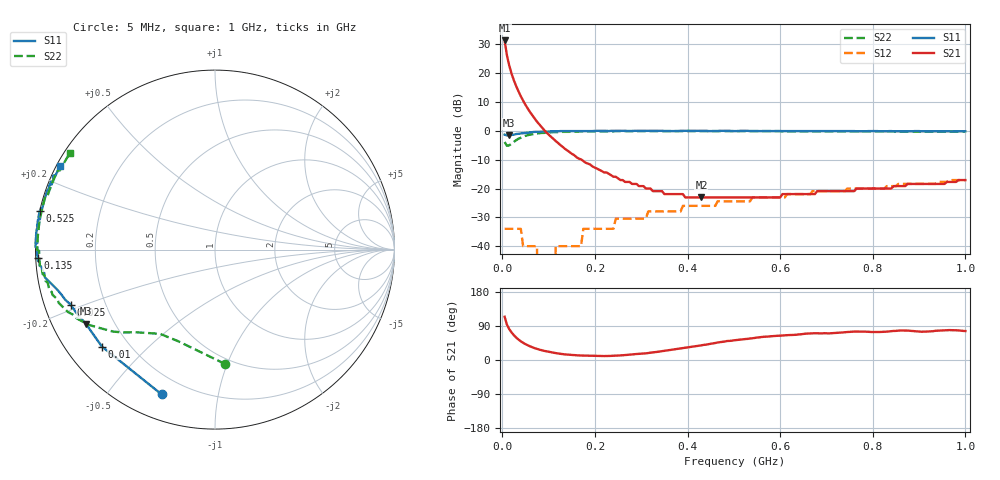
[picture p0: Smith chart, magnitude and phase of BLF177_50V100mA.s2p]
! Filename:  BLF177_50V100mA.s2p
! Philips part #: BLF177
!date: 21-05-2003
!Vdd=50V ; Idq=100mA
!D:\Vee measurements\measurement data\VDMOST\BLF177\50V_100mA_#1
# HZ S MA R 50
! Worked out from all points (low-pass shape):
!   200 points, 5 MHz to 1 GHz, reference 50 ohm
!   highest |S21| = 31.34 dB at 5 MHz (marker M1); lowest = -23.1 dB at 430 MHz (marker M2)
!   |S21| within 3 dB of the highest: start of sweep to 7.911 MHz
!   lowest |S11| = -1.6 dB at 15 MHz (marker M3), VSWR 10.76, Z = 4.97 - j13.2 ohm
!   |S11| at or under -10 dB: nowhere
!   |S22| runs from -5.2 to -0.1 dB; largest |S21 - S12| = 37
!   S11 on the Smith chart (normalised r, x): 5 MHz: 0.11, -0.69; 10 MHz: 0.11, -0.37; 25 MHz: 0.08, -0.18; 135 MHz: 0.01, -0.02; 525 MHz: -0.00, +0.11; 1 GHz: 0.01, +0.25
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5000000  0.86 -110.2  36.9 114.2  0.02 25.2  0.64 -84.9
1e7  0.83 -139.4  20.39 93.3  0.02 5.1  0.55 -112.0
1.5e7  0.83 -150.2  13.54 81.5  0.02 -5.7  0.56 -123.0
2e7  0.85 -155.7  9.82 72.6  0.02 -13.4  0.6 -129.3
2.5e7  0.86 -159.0  7.52 65.5  0.02 -19.6  0.64 -134.0
3.5e7  0.89 -163.4  4.82 53.9  0.02 -28.7  0.73 -141.3
4.5e7  0.91 -166.1  3.33 45.4  0.01 -34.1  0.79 -146.9
5.5e7  0.93 -168.1  2.43 38.8  0.01 -36.7  0.84 -151.5
7.5e7  0.96 -171.5  1.44 29.2  0.01 -29.7  0.9 -158.5
8e7  0.96 -172.2  1.29 27.4  0 -23.0  0.91 -159.9
1.1e8  0.98 -175.2  0.73 19.4  0 67.4  0.95 -166.4
1.15e8  0.98 -175.7  0.67 18.3  0.01 73.9  0.95 -167.3
1.35e8  0.99 -177.2  0.49 14.8  0.01 85.6  0.96 -170.1
1.7e8  0.99 -179.5  0.32 11.8  0.01 90.5  0.98 -174.0
1.75e8  0.99 -179.8  0.3 11.6  0.02 90.7  0.98 -174.5
3.4e8  1 173.7  0.09 22.4  0.04 88.4  0.99 174.8
4.3e8  1 170.8  0.07 38.7  0.05 87.3  0.99 170.5
5.05e8  0.99 168.4  0.07 52.6  0.06 86.3  0.99 167.2
5.25e8  1 167.7  0.07 55.3  0.06 86.2  0.99 166.3
6.7e8  0.99 163.2  0.08 70.4  0.09 84.5  0.98 160.2
8.35e8  0.99 157.8  0.1 75.4  0.11 84.5  0.98 153.4
1e9  0.98 151.8  0.14 76.4  0.14 79.8  0.97 146.2
